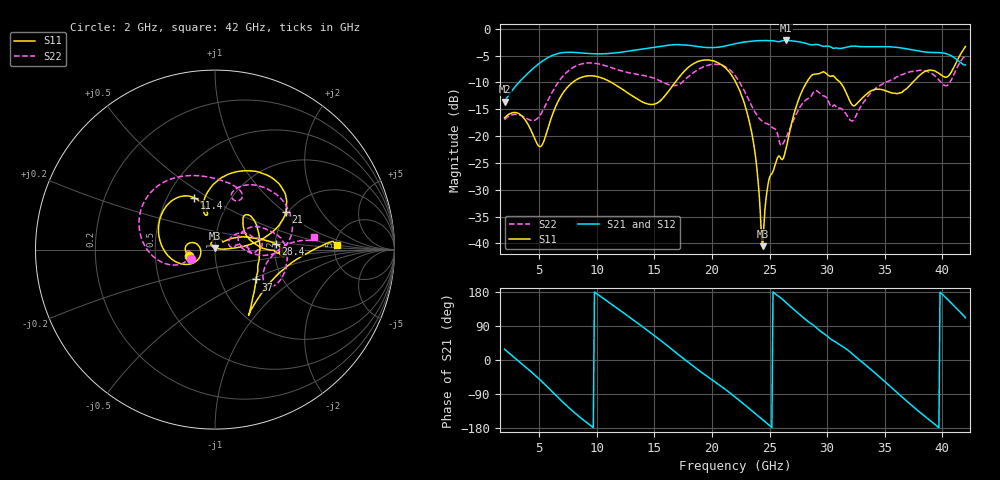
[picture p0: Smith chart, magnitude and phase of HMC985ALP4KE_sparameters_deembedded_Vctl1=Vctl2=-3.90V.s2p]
!s2p File: Measurements: S11, S21, S12, S22
# GHz S dB R 50.0
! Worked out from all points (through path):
!   401 points, 2 GHz to 42 GHz, reference 50 ohm
!   highest |S21| = -2.19 dB at 26.4 GHz (marker M1); lowest = -13.6 dB at 2 GHz (marker M2)
!   lowest |S11| = -40.5 dB at 24.4 GHz (marker M3), VSWR 1.02, Z = 50.1 + j0.941 ohm
!   |S11| at or under -10 dB: start of sweep to 7.907 GHz; 22.07 GHz to 28.22 GHz (6.145 GHz wide, 24.4 % of centre); 31.13 GHz to 37.42 GHz (6.294 GHz wide, 18.4 % of centre)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
!   |S22| runs from -21.8 to -5.1 dB; largest |S21 - S12| = 0.00061
!   S11 on the Smith chart (normalised r, x): 2 GHz: 0.75, -0.06; 11.4 GHz: 0.68, +0.44; 21 GHz: 1.95, +1.02; 28.4 GHz: 2.01, +0.15; 37 GHz: 1.48, -0.53; 42 GHz: 5.24, +0.46
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2  -16.60 -164.9  -13.60 28.4  -13.60 28.3  -16.96 -159.4
3.4  -16.09 169.2  -9.64 -7.7  -9.64 -7.7  -16.16 -177.0
5.1  -21.98 -172.6  -6.32 -53.0  -6.33 -53.0  -16.05 -160.9
6.3  -15.18 -151.8  -4.86 -88.5  -4.86 -88.5  -11.19 -162.8
8.7  -9.05 149.6  -4.52 -155.0  -4.52 -155.0  -6.55 150.6
11.4  -10.17 111.7  -4.56 144.5  -4.56 144.5  -7.34 106.2
13.6  -13.22 101.8  -3.92 96.1  -3.92 96.1  -8.54 75.4
15.4  -13.65 106.5  -3.33 55.1  -3.33 55.1  -9.63 62.6
17.9  -7.29 78.7  -3.08 -5.2  -3.08 -5.2  -9.03 71.4
21  -7.00 28.1  -3.29 -73.8  -3.29 -73.8  -6.90 16.8
22  -9.68 16.6  -2.82 -97.4  -2.82 -97.4  -8.71 -0.2
23.4  -18.85 4.9  -2.34 -132.3  -2.34 -132.3  -14.17 -5.1
24.4  -40.52 86.0  -2.21 -157.5  -2.21 -157.5  -17.31 9.1
25  -27.70 123.5  -2.24 -172.8  -2.24 -172.8  -17.93 12.4
26.4  -22.64 40.9  -2.19 152.4  -2.19 152.4  -20.41 33.9
28.4  -9.39 5.6  -2.89 100.2  -2.89 100.2  -12.97 17.2
28.7  -8.61 0.6  -3.02 94.1  -3.02 94.1  -12.24 15.5
32.4  -14.34 31.0  -3.25 10.4  -3.25 10.4  -16.66 27.1
35.4  -11.80 16.4  -3.37 -67.7  -3.37 -67.7  -9.73 18.1
37  -10.96 -35.9  -3.79 -110.8  -3.79 -110.8  -8.15 3.4
39.7  -8.31 -57.0  -4.46 -178.7  -4.46 -178.7  -9.55 -34.3
42  -3.33 2.0  -6.75 111.4  -6.75 111.4  -5.06 7.1
